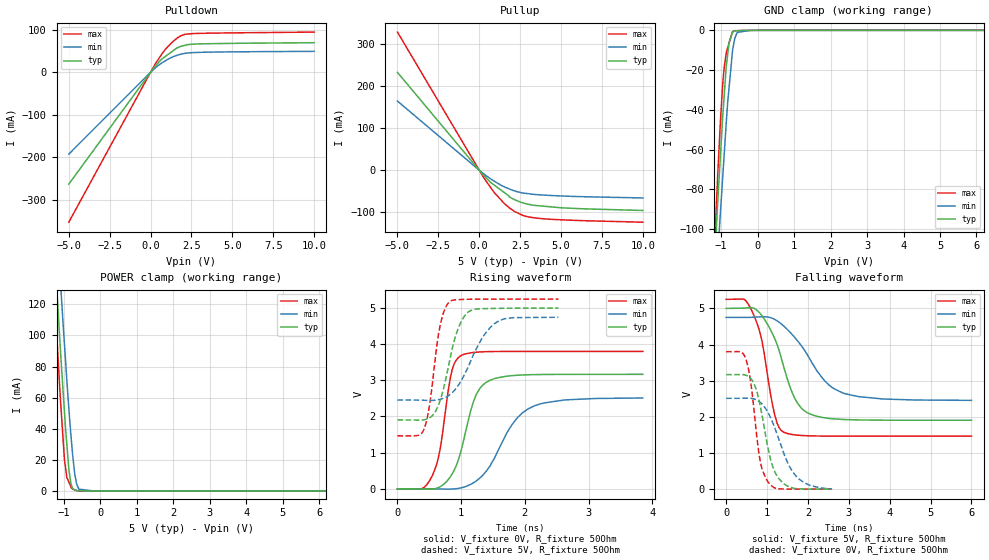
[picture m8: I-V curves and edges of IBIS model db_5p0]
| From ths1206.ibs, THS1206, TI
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|   db_5p0 Model
[Model]   db_5p0
Model_type   I/O
Polarity   Non-Inverting
Enable   Active-High
Vinl = 0.6
Vinh = 2.6
Vmeas = 2.5
Vref = 2.5
Cref = 30pF
Rref = 50
|   typ   min   max
|   (nom PVT)   (fast PVT)   (slow PVT)
C_comp   1.747e-12   1.743e-12   1.778e-12
|ON state : BUFFER OUTPUT TURNED HIGH
|C_comp   1.893e-12   1.893e-12   1.946e-12
|OFF state: BUFFER IN HIGH IMPEDANCE
|C_comp   1.601e-12   1.593e-12   1.609e-12
| Where nom  PVT is Nominal Process, 5V, 43C
|   Fast PVT is Strong Process,  5.25V, -55C
|   Slow PVT is Weak Process,   4.75V, 145C
[Voltage Range]   5   4.75   5.25
|Ambient Temperature   25   125   -55
|Junction Temperature
[Temperature Range]   43   145   -55
[Pullup Reference]   5   4.75   5.25
[Pulldown Reference]   0   0   0
[Power Clamp Reference]   5   4.75   5.25
[GND Clamp Reference]   0   0   0
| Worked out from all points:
|   slope of the pulldown table from 0 to 0.75 V, typ, clamps not added: 22.8 ohm
|   slope of the pullup table from 0 to 0.75 V, typ, clamps not added: 24.5 ohm
|   GND clamp passes 1 mA (typ) near -0.69 V on its own axis
|   POWER clamp passes 1 mA (typ) near -0.73 V on its own axis
|   falling waveform, V_fixture 5V, R_fixture 50Ohm: 20-80 % time 576ps typ, 880ps min, 372ps max; typ from 5 V to 1.91 V
|   rising waveform, V_fixture 0V, R_fixture 50Ohm: 20-80 % time 299ps typ, 509ps min, 200ps max; typ from 0 V to 3.17 V
|   rising waveform, V_fixture 5V, R_fixture 50Ohm: 20-80 % time 258ps typ, 401ps min, 172ps max; typ from 1.91 V to 5 V
|   falling waveform, V_fixture 0V, R_fixture 50Ohm: 20-80 % time 348ps typ, 542ps min, 247ps max; typ from 3.17 V to 0.001 V
[Pulldown]
|   Voltage   I(typ)   I(min)   I(max)
-5V       -263mA     -192.4mA   -352.4mA
283.5mV   14.1mA     10.08mA    19.52mA
700mV     31.51mA    22.11mA    43.39mA
924mV     37.8mA     27.28mA    54.61mA
1.286V    47.97mA    34.89mA    69.5mA
1.596V    56.66mA    39.65mA    79.62mA
1.827V    60.63mA    42.29mA    85.41mA
2.111V    63.43mA    44.54mA    89.26mA
2.594V    66.03mA    46.21mA    90.97mA
10V       69.5mA     49.19mA    94.44mA
[GND Clamp]
|   Voltage   I(typ)   I(min)   I(max)
-5V       -1.73A     -1.633A    -1.893A
-1.306V   -160.8mA   -182.5mA   -159.5mA
-1.092V   -85.92mA   -113.5mA   -72.03mA
-1.08V    -81.82mA   -109.8mA   -67.59mA
-1.031V   -66.39mA   -94.75mA   -49.77mA
-913.5mV  -32.08mA   -61.59mA   -18.22mA
-855mV    -17.29mA   -45.04mA   -10.86mA
-780mV    -5.877mA   -28.28mA   -6.223mA
-640.5mV  -377uA     -5.37mA    -190.7uA
-560.5mV  -239.7uA   -1.052mA   -166.9uA
-190mV    0A         -96.36nA   -56.58uA
10V       0A         0A         0A
[Pullup]
|   Voltage   I(typ)   I(min)   I(max)
-5V       232.7mA    164.4mA    328.5mA
294mV     -12.97mA   -9.238mA   -18.95mA
700mV     -29.21mA   -20.74mA   -41.41mA
924mV     -35.65mA   -26.23mA   -53.46mA
1.507V    -52.42mA   -39.06mA   -78.24mA
1.822V    -61.48mA   -44.32mA   -88.88mA
1.833V    -63.34mA   -44.5mA    -89.18mA
2.14V     -69.74mA   -49.03mA   -97.68mA
2.678V    -77.87mA   -54.31mA   -107.9mA
3.365V    -83.58mA   -57.64mA   -113.3mA
5.405V    -90.19mA   -61.86mA   -118.6mA
10V       -95.75mA   -66.04mA   -123.7mA
[POWER Clamp]
|   Voltage   I(typ)   I(min)   I(max)
-5V       1.847A     1.834A     1.872A
-1.306V   174.9mA    216.9mA    147.2mA
-1.103V   94.46mA    138.3mA    62.29mA
-1.08V    85.66mA    129.8mA    54.37mA
-981.8mV  50.45mA    93.94mA    20.18mA
-918.7mV  30.35mA    71.69mA    8.72mA
-860mV    13.62mA    52.29mA    5.584mA
-805mV    4.702mA    35.81mA    2.648mA
-698.3mV  670.3uA    10.7mA     592.5uA
-589mV    110.3uA    1.142mA    119uA
-190mV    0A         26.4nA     2.328uA
10V       0A         0A         0A
[Ramp]
R_load = 50
|   typ   min   max
dV/dt_r   1.90032/2.98059e-10   1.50742/5.05845e-10   2.28107/1.99197e-10
dV/dt_f   1.85642/5.76124e-10   1.37608/8.78103e-10   2.27014/3.70788e-10
[Falling Waveform]
V_fixture = 5V
V_fixture_min = 4.75V
V_fixture_max = 5.25V
R_fixture = 50Ohm
|   Time   V(typ)   V(min)   V(max)
0s        5V         4.75V      5.25V
436ps     5.006V     4.749V     5.258V
674ps     5.005V     4.756V     4.82V
874ps     4.8V       4.768V     4.114V
1.192ns   4.155V     4.693V     2.041V
1.4ns     3.418V     4.521V     1.583V
1.848ns   2.233V     3.955V     1.485V
2.388ns   1.977V     3.024V     1.469V
2.85ns    1.928V     2.661V     1.467V
6ns       1.906V     2.457V     1.466V
[Rising Waveform]
V_fixture = 0V
V_fixture_min = 0V
V_fixture_max = 0V
R_fixture = 50Ohm
|   Time   V(typ)   V(min)   V(max)
0s        1.91nV     4.517nV    1.571nV
546ps     -9.673mV   -2.061mV   361.1mV
664ps     51.14mV    -5.568mV   1.048V
856ps     402.8mV    -7.524mV   3.273V
986ps     972.6mV    20.35mV    3.671V
1.232ns   2.587V     210.5mV    3.778V
1.452ns   3.001V     628.9mV    3.796V
1.8ns     3.131V     1.777V     3.801V
2.16ns    3.159V     2.301V     3.801V
3.852ns   3.167V     2.512V     3.802V
[Rising Waveform]
V_fixture = 5V
V_fixture_min = 4.75V
V_fixture_max = 5.25V
R_fixture = 50Ohm
|   Time   V(typ)   V(min)   V(max)
0s        1.906V     2.455V     1.466V
418ps     1.909V     2.449V     1.652V
510ps     1.969V     2.445V     2.389V
672ps     2.456V     2.476V     4.536V
830ps     3.635V     2.613V     5.19V
954ps     4.441V     2.859V     5.235V
1.098ns   4.873V     3.325V     5.244V
1.318ns   4.982V     4.136V     5.248V
1.524ns   4.991V     4.571V     5.249V
2.528ns   5V         4.746V     5.25V
[Falling Waveform]
V_fixture = 0V
V_fixture_min = 0V
V_fixture_max = 0V
R_fixture = 50Ohm
|   Time   V(typ)   V(min)   V(max)
0s        3.167V     2.513V     3.802V
362ps     3.17V      2.514V     3.791V
488ps     3.15V      2.516V     3.578V
604ps     3.058V     2.512V     2.937V
808ps     2.441V     2.424V     944.6mV
904ps     1.884V     2.322V     476.5mV
1.03ns    1.105V     2.107V     194.3mV
1.274ns   314.5mV    1.43V      10.18mV
1.684ns   19.33mV    395.6mV    1.376mV
2.59ns    837.9uV    6.35mV     207.7uV
